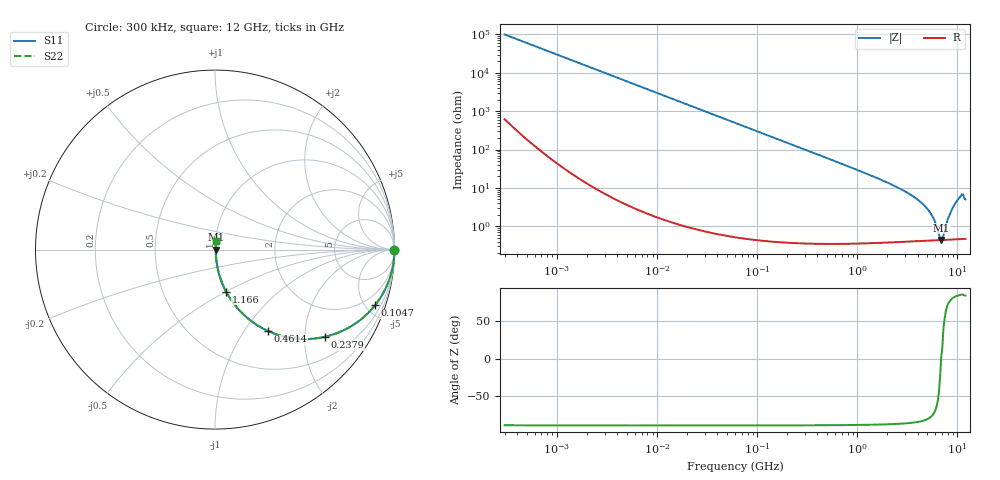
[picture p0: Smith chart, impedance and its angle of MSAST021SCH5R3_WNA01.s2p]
! MSAST021SCH5R3_WNA01  S-PARAMETER MODEL  ( General Type )
! Model Generated by TAIYO YUDEN Corporation (http://www.ty-top.com)
! Version 2.0
! TAIYO YUDEN Control No. 181101
! Copyright(c) 2015 TAIYO YUDEN CO.,LTD. All Rights Reserved.
! Product Description (link to TY-COMPAS)
! https://ds.yuden.co.jp/TYCOMPAS/or/detail?pn=MSAST021SCH5R3CWNA01&u=M
! Products Name : Multilayer Ceramic Capacitors
! Characteristics :
!  Capacitance : 5.3 pF , Rated Voltage : 25V , TCC : CH / C0H
!  Case Size : 0.25 x 0.125 / 0.0098 x 0.0049 [mm/inch] , Thickness : 0.125 / 0.0049 [mm/inch]
!  (Conditions: Temperature = 25 degC , DC Bias Current/Voltage = 0A / 0V)
! External Node Assignments :
!  1  o---| |---o  2
! GND o---------o GND
! Frequency Range : 0.3MHz  -  12000MHz  [ 401 STEP ]
# MHz S RI R 50
! Freq[MHz].  S11 Real  S11 Imag  S21 Real  S21 Imag  S12 Real  S12 Imag  S22 Real  S22 Imag
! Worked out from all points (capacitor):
!   401 points, 300 kHz to 12 GHz, reference 50 ohm
!   read as one part in series: C = 5.3 pF near 316.3 kHz
!   lowest |Z| = 440 mohm at 6.88 GHz (marker M1)
!   series resonance near 6.871 GHz, so ESL is about 100 pH
!   S11 on the Smith chart (normalised r, x): 300 kHz: open; 104.7 MHz: 1.01, -5.74; 237.9 MHz: 1.01, -2.52; 461.4 MHz: 1.01, -1.30; 1.166 GHz: 1.01, -0.50; 12 GHz: 1.01, +0.10
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0.3  1 -0.000999  7.13e-06 0.000999  7.13e-06 0.000999  1 -0.000999
1.769972  1 -0.00589  4.02e-05 0.00589  4.02e-05 0.00589  1 -0.00589
10.44266  0.9988 -0.0347  0.00123 0.0347  0.00123 0.0347  0.9988 -0.0347
60  0.9614 -0.1921  0.0386 0.1921  0.0386 0.1921  0.9614 -0.1921
104.6549  0.8913 -0.3105  0.1087 0.3105  0.1087 0.3105  0.8913 -0.3105
237.9135  0.6135 -0.4855  0.3865 0.4855  0.3865 0.4855  0.6135 -0.4855
353.9943  0.4175 -0.4911  0.5825 0.4911  0.5825 0.4911  0.4175 -0.4911
461.3684  0.2967 -0.4541  0.7033 0.4541  0.7033 0.4541  0.2967 -0.4541
723.8279  0.1462 -0.3491  0.8538 0.3491  0.8538 0.3491  0.1462 -0.3491
1166.079  0.0618 -0.2338  0.9382 0.2338  0.9382 0.2338  0.0618 -0.2338
2088.533  0.0203 -0.1273  0.9797 0.1273  0.9797 0.1273  0.0203 -0.1273
3364.605  0.00851 -0.067  0.9915 0.067  0.9915 0.067  0.00851 -0.067
4623.766  0.0054 -0.0351  0.9946 0.0351  0.9946 0.0351  0.0054 -0.0351
5565.855  0.0046 -0.0183  0.9954 0.0183  0.9954 0.0183  0.0046 -0.0183
6026.253  0.00443 -0.0113  0.9956 0.0113  0.9956 0.0113  0.00443 -0.0113
6524.734  0.00437 -0.00438  0.9956 0.00438  0.9956 0.00438  0.00437 -0.00438
6879.757  0.00437 0.000107  0.9956 -0.000107  0.9956 -0.000107  0.00437 0.000107
7254.098  0.00442 0.00384  0.9956 -0.00384  0.9956 -0.00384  0.00442 0.00384
8281.503  0.0048 0.018  0.9952 -0.018  0.9952 -0.018  0.0048 0.018
9454.42  0.00598 0.0378  0.994 -0.0378  0.994 -0.0378  0.00598 0.0378
10793.46  0.00827 0.0602  0.9917 -0.0602  0.9917 -0.0602  0.00827 0.0602
12000  0.00712 0.0493  0.9929 -0.0493  0.9929 -0.0493  0.00712 0.0493
